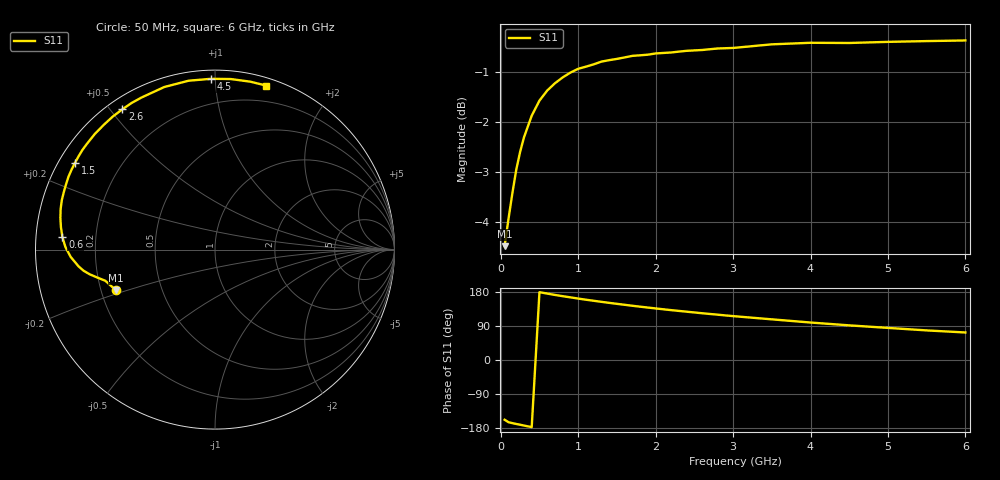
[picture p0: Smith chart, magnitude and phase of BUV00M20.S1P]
! Infineon Technologies  Discrete & RF Semiconductors
! BB 833
! Si Tuning Diode in SOD323
! VR =
! S-Parameters:  June  1999
# GHz  S  MA  R  50
!  f  S11
! GHz  MAG  ANG
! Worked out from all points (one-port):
!   34 points, 50 MHz to 6 GHz, reference 50 ohm
!   lowest |S11| = -4.5 dB at 50 MHz (marker M1), VSWR 3.95, Z = 13.1 - j9.24 ohm
!   |S11| at or under -10 dB: nowhere
!   S11 on the Smith chart (normalised r, x): 50 MHz: 0.26, -0.18; 600 MHz: 0.08, +0.04; 1.5 GHz: 0.05, +0.28; 2.6 GHz: 0.04, +0.54; 4.5 GHz: 0.05, +0.97; 6 GHz: 0.06, +1.36
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0.05  0.5962 -157.6
0.1  0.6348 -164.1
0.2  0.7107 -168.8
0.25  0.7407 -170.8
0.3  0.766 -173.0
0.4  0.8051 -177.1
0.5  0.8336 179.0
0.6  0.8531 175.3
0.7  0.8676 171.7
0.8  0.8794 168.4
0.9  0.8892 165.3
1.1  0.9014 159.1
1.3  0.9119 153.5
1.5  0.9176 148.2
1.6  0.9208 145.7
1.7  0.9241 143.1
2  0.9292 136.1
2.2  0.9313 131.6
2.4  0.9349 127.5
2.6  0.9366 123.4
2.8  0.9399 119.6
3  0.9411 115.8
3.5  0.9489 107.3
4  0.9523 98.9
4.5  0.9519 91.4
5  0.9543 84.7
5.5  0.956 78.1
6  0.9574 72.6
